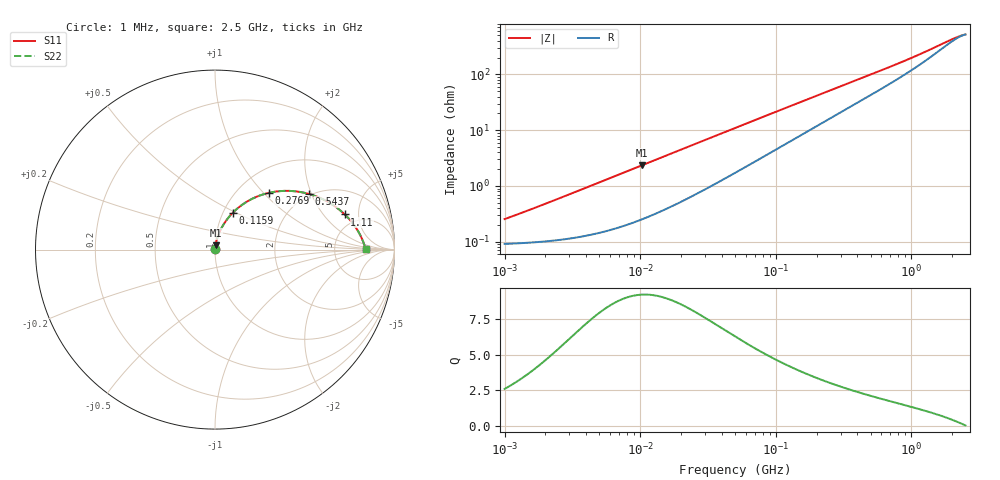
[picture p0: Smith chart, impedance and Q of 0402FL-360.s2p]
# MHz S MA R 50
!Freq  MagS11  AngS11  MagS21  AngS21  MagS12  AngS12  MagS22  AngS22
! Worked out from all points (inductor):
!   801 points, 1 MHz to 2.5 GHz, reference 50 ohm
!   read as one part in series: L = 37.6 nH near 1.181 MHz
!   highest Q = 9.25 at 10.35 MHz (marker M1), where L = 36.1 nH
!   S11 on the Smith chart (normalised r, x): 1 MHz: 1.00, +0.00; 115.9 MHz: 1.11, +0.48; 276.9 MHz: 1.37, +1.07; 543.7 MHz: 1.96, +1.93; 1.11 GHz: 3.81, +3.40; 2.5 GHz: 11, +0
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1  0.002545 68.8  0.9991 -0.1  0.9991 -0.1  0.002545 68.8
1.081383  0.002725 70.1  0.9991 -0.1  0.9991 -0.1  0.002725 70.1
1.568128  0.003818 75.1  0.999 -0.2  0.999 -0.2  0.003818 75.1
3.70813  0.008671 81.3  0.9987 -0.5  0.9987 -0.5  0.008671 81.3
10.35463  0.02353 82.5  0.9972 -1.3  0.9972 -1.3  0.02353 82.5
13.61641  0.0307 82.0  0.9962 -1.7  0.9962 -1.7  0.0307 82.0
27.53449  0.06064 79.3  0.9905 -3.4  0.9905 -3.4  0.06064 79.3
50  0.1069 74.9  0.9777 -6.1  0.9777 -6.1  0.1069 74.9
79.17699  0.1631 69.9  0.9562 -9.2  0.9562 -9.2  0.1631 69.9
115.9441  0.2276 64.3  0.9242 -12.8  0.9242 -12.8  0.2276 64.3
146.6178  0.2761 60.1  0.8952 -15.5  0.8952 -15.5  0.2761 60.1
185.4065  0.3308 55.5  0.8572 -18.5  0.8572 -18.5  0.3308 55.5
276.8658  0.4348 46.6  0.7691 -24.2  0.7691 -24.2  0.4348 46.6
389.8785  0.5264 38.4  0.6725 -29.1  0.6725 -29.1  0.5264 38.4
543.6779  0.6098 30.5  0.5667 -33.1  0.5667 -33.1  0.6098 30.5
680.8203  0.66 25.4  0.4929 -35.0  0.4929 -35.0  0.66 25.4
869.3969  0.708 20.1  0.4142 -36.0  0.4142 -36.0  0.708 20.1
1110.206  0.7489 15.2  0.3395 -35.3  0.3395 -35.3  0.7489 15.2
1518.173  0.7916 9.3  0.2533 -30.3  0.2533 -30.3  0.7916 9.3
2096.459  0.825 3.4  0.1833 -15.7  0.1833 -15.7  0.825 3.4
2334.576  0.8338 1.5  0.1679 -7.4  0.1679 -7.4  0.8338 1.5
2500  0.8387 0.2  0.1613 -1.2  0.1613 -1.2  0.8387 0.2
